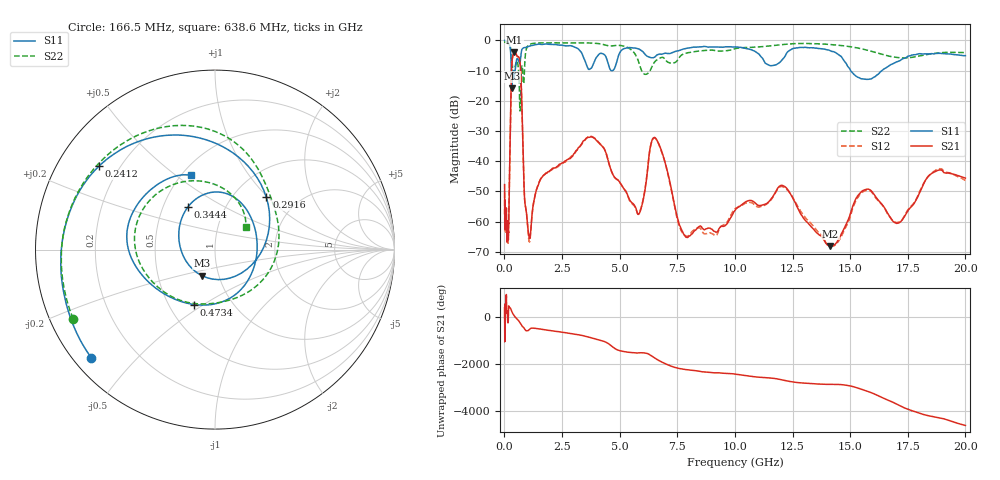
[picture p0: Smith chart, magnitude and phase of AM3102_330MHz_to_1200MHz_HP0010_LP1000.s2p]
! Date/Time: Tue, Sep 11, 2018 5:11 PM
! Network Analyzer: Agilent Technologies E8362B Rev: A.07.50.63
! Sweep from 0.010 to 20.000 GHz, 1601 Points, Sweep Type: LOG
! Power Supply: 4.949 V, 0.001 A
# Hz S DB R 50
!freq MagS11 AngS11 MagS21 AngS21 MagS12 AngS12 MagS22 AngS22
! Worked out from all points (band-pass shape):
!   1601 points, 10 MHz to 20 GHz, reference 50 ohm
!   highest |S21| = -3.92 dB at 432.6 MHz (marker M1); lowest = -68.0 dB at 14.14 GHz (marker M2)
!   |S21| within 3 dB of the highest: 331.7 MHz to 674.9 MHz (343.3 MHz wide, 68.2 % of centre)
!   lowest |S11| = -15.8 dB at 319.2 MHz (marker M3), VSWR 1.39, Z = 41.5 - j12.4 ohm
!   |S11| at or under -10 dB: 298.2 MHz to 355.5 MHz (57.32 MHz wide, 17.5 % of centre); 369.1 MHz to 467.8 MHz (98.74 MHz wide, 23.6 % of centre); 15.03 GHz to 16.38 GHz (1.352 GHz wide, 8.61 % of centre)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
!   |S22| runs from -23.4 to -0.3 dB; largest |S21 - S12| = 0.012
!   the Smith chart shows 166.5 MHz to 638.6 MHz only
!   S11 on the Smith chart (normalised r, x): 166.5 MHz: 0.05, -0.38; 241.2 MHz: 0.12, +0.32; 291.6 MHz: 1.40, +0.98; 344.4 MHz: 0.67, +0.35; 473.4 MHz: 0.67, -0.46; 638.6 MHz: 0.55, +0.57
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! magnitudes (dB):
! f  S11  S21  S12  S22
! 10 MHz  0.0  -47.7  -50.4  -0.3
! 35.55 MHz  0.0  -60.5  -61.3  -0.5
! 126.4 MHz  -0.4  -62.0  -63.6  -0.9
! 166.5 MHz  -0.8  -64.2  -64.6  -1.1
! 241.2 MHz  -2.0  -37.0  -37.0  -1.8
! 291.6 MHz  -7.8  -15.4  -15.5  -3.6
! 319.2 MHz  -15.8  -8.4  -8.4  -6.4
! 344.4 MHz  -11.0  -6.1  -6.1  -8.3
! 432.6 MHz  -11.9  -3.9  -4.0  -10.0
! 447.2 MHz  -11.0  -3.9  -4.0  -9.4
! 473.4 MHz  -9.7  -4.1  -4.1  -8.4
! 638.6 MHz  -7.2  -5.7  -5.8  -13.5
! 873.8 MHz  -2.3  -51.9  -52.1  -9.3
! 1.067 GHz  -1.9  -64.9  -66.0  -1.4
! 1.59 GHz  -1.3  -45.6  -45.7  -0.8
! 3.775 GHz  -9.1  -31.9  -31.8  -0.9
! 5.652 GHz  -2.5  -54.7  -55.0  -4.3
! 6.58 GHz  -5.1  -32.6  -32.7  -6.6
! 7.882 GHz  -2.6  -65.2  -64.8  -4.2
! 12.03 GHz  -6.6  -48.0  -48.4  -1.4
! 14.14 GHz  -3.4  -68.0  -68.0  -1.3
! 20 GHz  -5.0  -45.6  -46.4  -4.0
